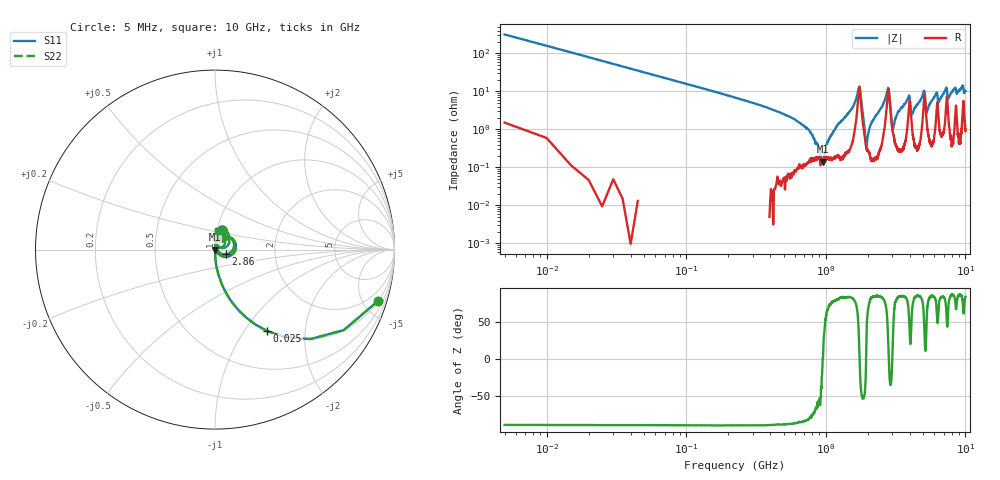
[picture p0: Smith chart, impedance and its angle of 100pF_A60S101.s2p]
! Amotech Co.,Ltd.
! http://www.amotech.co.kr/
! Part Number: A60S101
! These Parameters are Measured in Series Mode Connection
! Operation Temp=25[degC], DC Bias Voltage=0[V]
! Freq. Start=5[MHz] Stop=10[GHz], 2000[Steps]
! Date: Monday, July 13, 2020, 01:45:01
# GHZ S RI R 50.000000
!Freq.(Hz) S11(Real) S11(Imag) S21(Real) S21(Imag) S12(Real) S12(Imag) S22(Real) S22(Imag)
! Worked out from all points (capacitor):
!   2000 points, 5 MHz to 10 GHz, reference 50 ohm
!   read as one part in series: C = 99 pF near 55 MHz
!   lowest |Z| = 142 mohm at 955 MHz (marker M1)
!   series resonance near 949.4 MHz, so ESL is about 280 pH
!   S11 on the Smith chart (normalised r, x): 5 MHz: 1.03, -6.32; 25 MHz: 1.00, -1.28; 2.86 GHz: 1.13, -0.06; 10 GHz: 1.02, +0.21
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0.005  0.9079 -0.2868  0.0921 0.2868  0.0921 0.2868  0.9079 -0.2868
0.025  0.2906 -0.4539  0.7094 0.4539  0.7094 0.4539  0.2906 -0.4539
0.115  0.0182 -0.1361  0.9818 0.1361  0.9818 0.1361  0.0182 -0.1361
0.73  0.00134 -0.0105  0.9987 0.0105  0.9987 0.0105  0.00134 -0.0105
0.955  0.00142 2.51e-05  0.9986 -2.51e-05  0.9986 -2.51e-05  0.00142 2.51e-05
1.175  0.00212 0.0108  0.9979 -0.0108  0.9979 -0.0108  0.00212 0.0108
1.675  0.0335 0.0681  0.9665 -0.0681  0.9665 -0.0681  0.0335 0.0681
1.765  0.0836 -0.0359  0.9164 0.0359  0.9164 0.0359  0.0836 -0.0359
1.96  0.0032 0.00207  0.9968 -0.00207  0.9968 -0.00207  0.0032 0.00207
2.125  0.00172 0.0152  0.9983 -0.0152  0.9983 -0.0152  0.00172 0.0152
2.765  0.0729 0.0723  0.9271 -0.0723  0.9271 -0.0723  0.0729 0.0723
2.86  0.0618 -0.0265  0.9382 0.0265  0.9382 0.0265  0.0618 -0.0265
3.02  0.00854 0.00446  0.9915 -0.00446  0.9915 -0.00446  0.00854 0.00446
3.34  0.00377 0.0304  0.9962 -0.0304  0.9962 -0.0304  0.00377 0.0304
3.94  0.0408 0.0614  0.9592 -0.0614  0.9592 -0.0614  0.0408 0.0614
4.135  0.0125 0.0219  0.9875 -0.0219  0.9875 -0.0219  0.0125 0.0219
5.005  0.0414 0.0807  0.9586 -0.0807  0.9586 -0.0807  0.0414 0.0807
5.265  0.0183 0.0198  0.9817 -0.0198  0.9817 -0.0198  0.0183 0.0198
6.19  0.0321 0.0826  0.9679 -0.0826  0.9679 -0.0826  0.0321 0.0826
6.67  0.0118 0.0666  0.9882 -0.0666  0.9882 -0.0666  0.0118 0.0666
8.335  0.0223 0.1135  0.9777 -0.1135  0.9777 -0.1135  0.0223 0.1135
10  0.0192 0.1009  0.9808 -0.1009  0.9808 -0.1009  0.0192 0.1009
